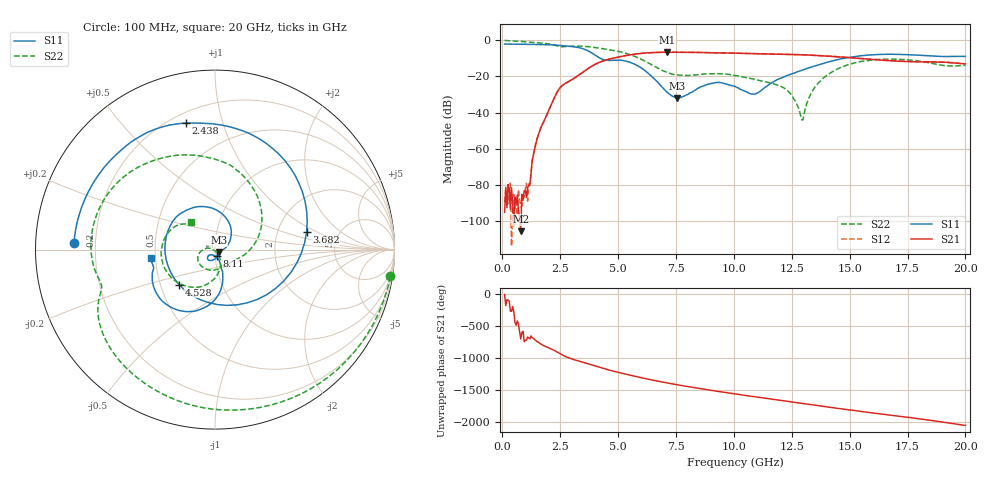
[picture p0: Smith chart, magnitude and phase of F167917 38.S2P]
!  2-Port S-parameters saved by WinCal
! VAR MeasName=S-Parameters (CALIBRATED_DATA) read from VNA (N5242A)
! VAR MeasDate=2016-11-22 9:01:38
! VAR NAME=F167917 38
! VAR FILENAME=F167917 38.S2P
! VAR DATE=2016-11-22 9:01:38
! VAR PHYS_PORTS=1,2
# Hz S DB R 50
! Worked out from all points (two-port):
!   401 points, 100 MHz to 20 GHz, reference 50 ohm
!   highest |S21| = -6.58 dB at 7.115 GHz (marker M1); lowest = -105.5 dB at 796.5 MHz (marker M2)
!   |S21| within 3 dB of the highest: 4.927 GHz to 14.94 GHz (10.01 GHz wide, 101 % of centre)
!   lowest |S11| = -31.8 dB at 7.562 GHz (marker M3), VSWR 1.05, Z = 52.1 - j1.61 ohm
!   |S11| at or under -10 dB: 4.236 GHz to 14.74 GHz (10.5 GHz wide, 111 % of centre)
!   |S22| runs from -44.1 to -0.1 dB; largest |S21 - S12| = 0.0058
!   S11 on the Smith chart (normalised r, x): 100 MHz: 0.12, +0.02; 2.438 GHz: 0.26, +0.76; 3.682 GHz: 2.93, +0.78; 4.528 GHz: 0.62, -0.26; 8.11 GHz: 1.02, -0.07; 20 GHz: 0.47, -0.05
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1e8  -2.09 177.3  -95.10 -13.0  -89.50 -65.4  -0.10 -8.7
7.965e8  -2.19 158.8  -105.51 12.8  -92.09 -167.6  -0.63 -63.3
1.14475e9  -2.25 149.1  -80.54 29.1  -79.47 46.6  -0.97 -87.5
1.5925e9  -2.35 135.7  -50.97 -48.2  -50.84 -48.3  -1.46 -115.7
2.43825e9  -2.81 103.0  -27.23 155.7  -27.24 155.4  -3.38 -159.7
3.43325e9  -4.49 38.4  -18.12 15.6  -18.14 15.7  -3.28 161.5
3.682e9  -5.69 10.7  -15.85 -10.9  -15.85 -10.7  -3.50 149.6
4.12975e9  -9.21 -59.0  -12.54 -60.9  -12.49 -60.8  -4.23 128.5
4.52775e9  -11.05 -135.7  -10.74 -102.8  -10.68 -103.0  -5.02 110.2
5.62225e9  -12.68 94.3  -7.86 160.0  -7.86 159.7  -8.39 51.8
6.7665e9  -23.99 12.4  -6.64 71.8  -6.66 71.8  -15.77 -11.0
7.11475e9  -28.67 -8.3  -6.58 47.7  -6.60 47.8  -17.76 -25.8
7.5625e9  -31.83 -37.1  -6.59 18.6  -6.61 18.6  -19.15 -44.5
8.10975e9  -28.99 -69.3  -6.61 -15.3  -6.61 -15.3  -19.35 -70.5
1.005e10  -25.45 -136.8  -7.12 -123.8  -7.13 -123.8  -19.48 -153.9
1.089575e10  -29.74 -101.2  -7.39 -167.6  -7.38 -167.6  -21.60 -171.1
1.21395e10  -20.38 -69.5  -7.76 129.3  -7.74 129.3  -26.13 171.3
1.29355e10  -16.57 -73.1  -8.02 88.9  -8.00 89.1  -44.05 -137.4
1.338325e10  -14.67 -76.6  -8.28 66.1  -8.24 66.4  -28.28 -58.6
1.4627e10  -10.28 -95.3  -9.27 4.5  -9.18 4.5  -15.00 -96.3
1.67165e10  -7.74 -136.2  -11.23 -93.4  -11.19 -93.9  -10.41 -169.3
2e10  -8.90 -172.8  -13.06 104.2  -13.01 103.7  -13.83 131.4
